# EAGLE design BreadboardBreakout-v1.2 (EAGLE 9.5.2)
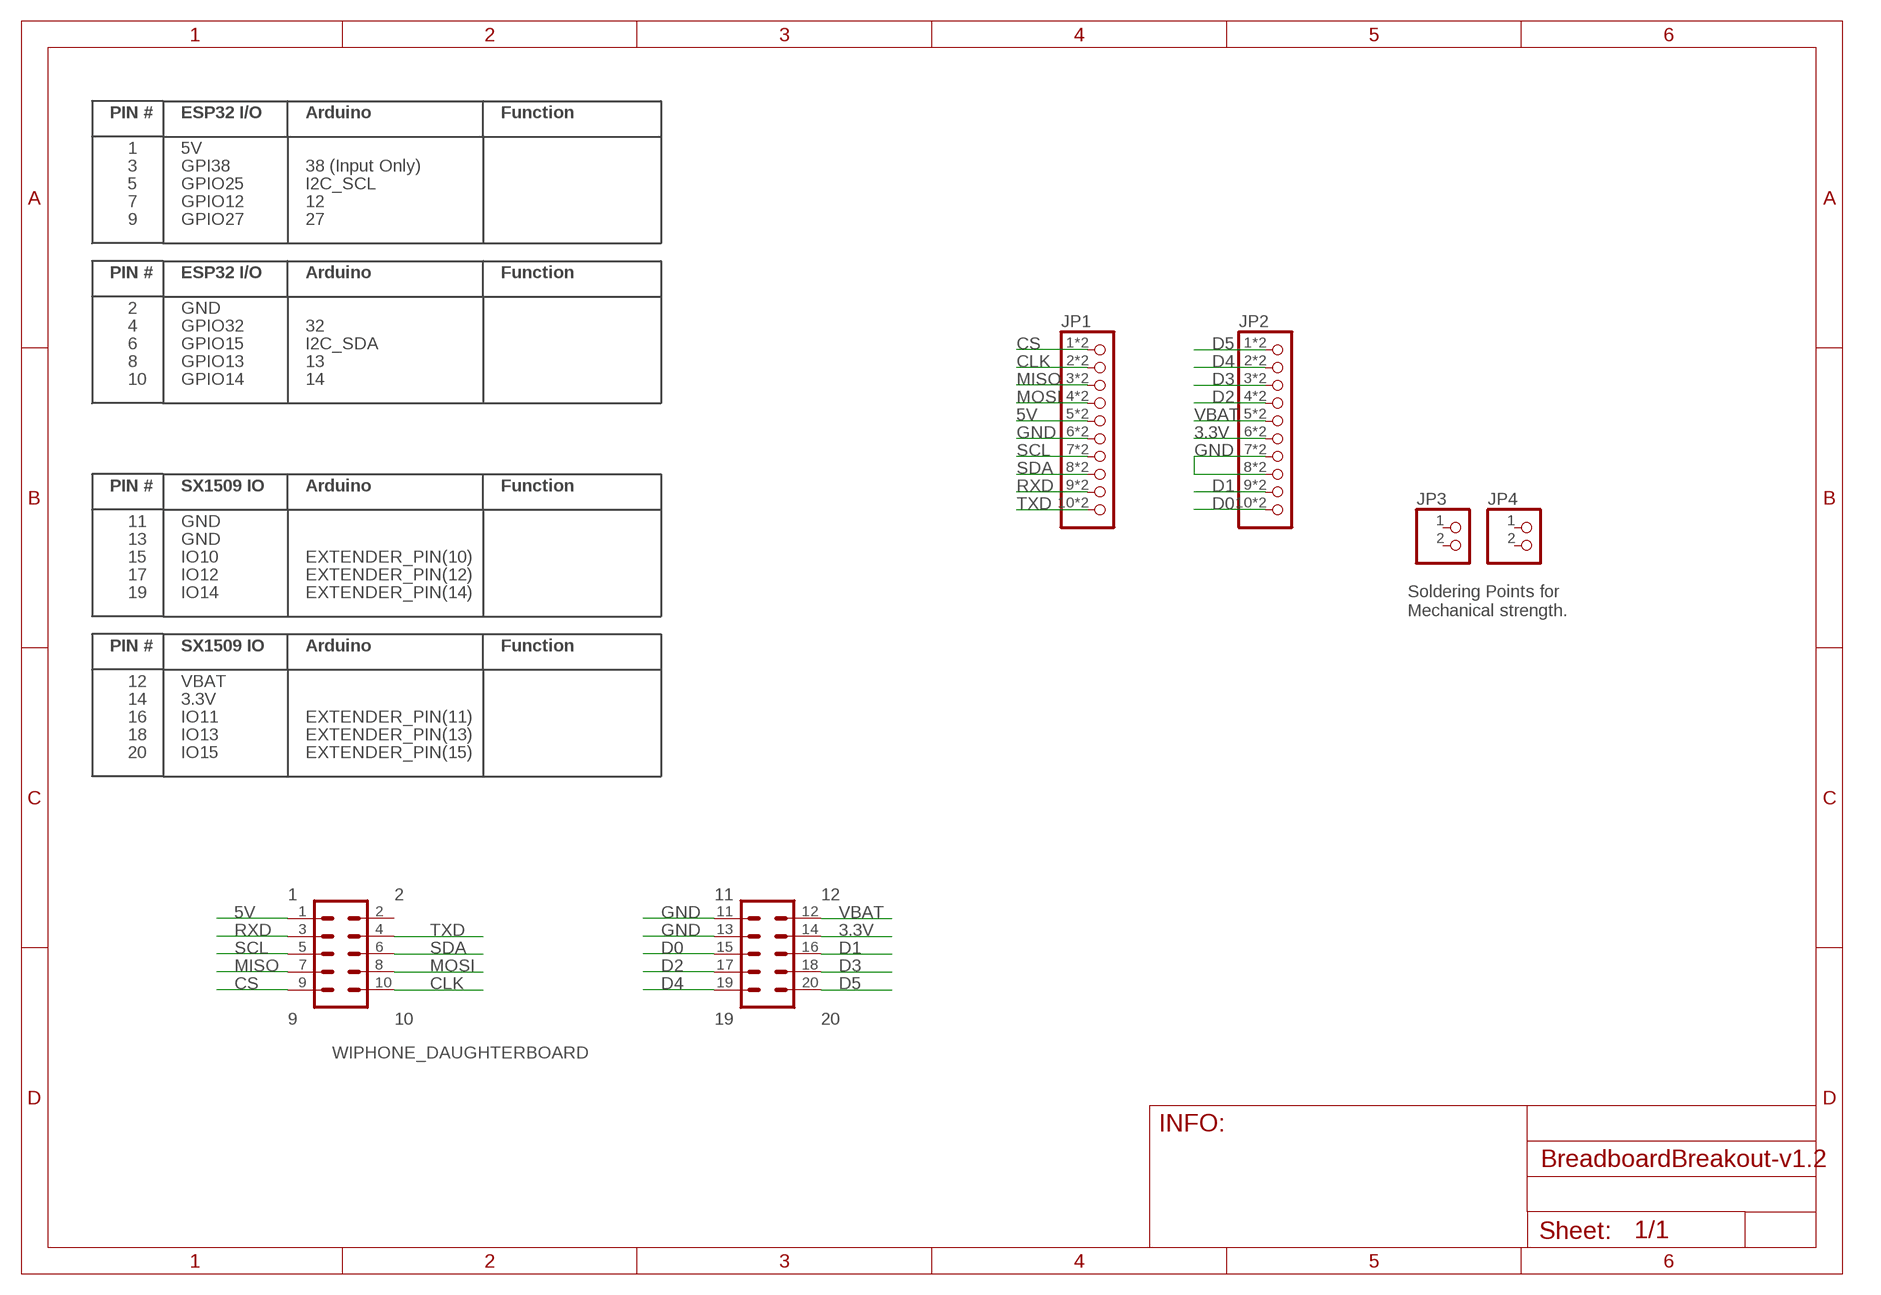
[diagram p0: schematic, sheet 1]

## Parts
JP1  PINHD-1X10_TH/SMD  [1X10TH/SMD]
JP2  PINHD-1X10_TH/SMD  [1X10TH/SMD]
JP3  PINHD-1X2_EXT  [1X02TH/EXT]
JP4  PINHD-1X2_EXT  [1X02TH/EXT]
WIPHONE_DAUGHTERBOARD-FOOTPRINT1  WIPHONE_DAUGHTERBOARD  [WIPHONE_DAUGHTERBOARD]

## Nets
3.3V: JP2.6 JP2.6P WIPHONE_DAUGHTERBOARD-FOOTPRINT1.14
5V: JP1.5 JP1.5P WIPHONE_DAUGHTERBOARD-FOOTPRINT1.1
CLK: JP1.2 JP1.2P WIPHONE_DAUGHTERBOARD-FOOTPRINT1.10
CS: JP1.1 JP1.1P WIPHONE_DAUGHTERBOARD-FOOTPRINT1.9
D0: JP2.10 JP2.10P WIPHONE_DAUGHTERBOARD-FOOTPRINT1.15
D1: JP2.9 JP2.9P WIPHONE_DAUGHTERBOARD-FOOTPRINT1.16
D2: JP2.4 JP2.4P WIPHONE_DAUGHTERBOARD-FOOTPRINT1.17
D3: JP2.3 JP2.3P WIPHONE_DAUGHTERBOARD-FOOTPRINT1.18
D4: JP2.2 JP2.2P WIPHONE_DAUGHTERBOARD-FOOTPRINT1.19
D5: JP2.1 JP2.1P WIPHONE_DAUGHTERBOARD-FOOTPRINT1.20
GND: JP1.6 JP1.6P JP2.7 JP2.7P JP2.8 JP2.8P WIPHONE_DAUGHTERBOARD-FOOTPRINT1.11 WIPHONE_DAUGHTERBOARD-FOOTPRINT1.13
MISO: JP1.3 JP1.3P WIPHONE_DAUGHTERBOARD-FOOTPRINT1.7
MOSI: JP1.4 JP1.4P WIPHONE_DAUGHTERBOARD-FOOTPRINT1.8
RXD: JP1.9 JP1.9P WIPHONE_DAUGHTERBOARD-FOOTPRINT1.3
SCL: JP1.7 JP1.7P WIPHONE_DAUGHTERBOARD-FOOTPRINT1.5
SDA: JP1.8 JP1.8P WIPHONE_DAUGHTERBOARD-FOOTPRINT1.6
TXD: JP1.10 JP1.10P WIPHONE_DAUGHTERBOARD-FOOTPRINT1.4
VBAT: JP2.5 JP2.5P WIPHONE_DAUGHTERBOARD-FOOTPRINT1.12
Unconnected: JP3.1 JP3.2 JP4.1 JP4.2

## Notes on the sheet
- Soldering Points for 
  Mechanical strength.

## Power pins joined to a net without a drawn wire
2: WIPHONE_DAUGHTERBOARD-FOOTPRINT1.2

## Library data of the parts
JP1 JP2 = WiPhone:PINHD-1X10: PIN HEADER
JP3 JP4 = WiPhone:PINHD-1X2: PIN HEADER
WIPHONE_DAUGHTERBOARD-FOOTPRINT1 = WiPhone:WIPHONE_DAUGHTERBOARD

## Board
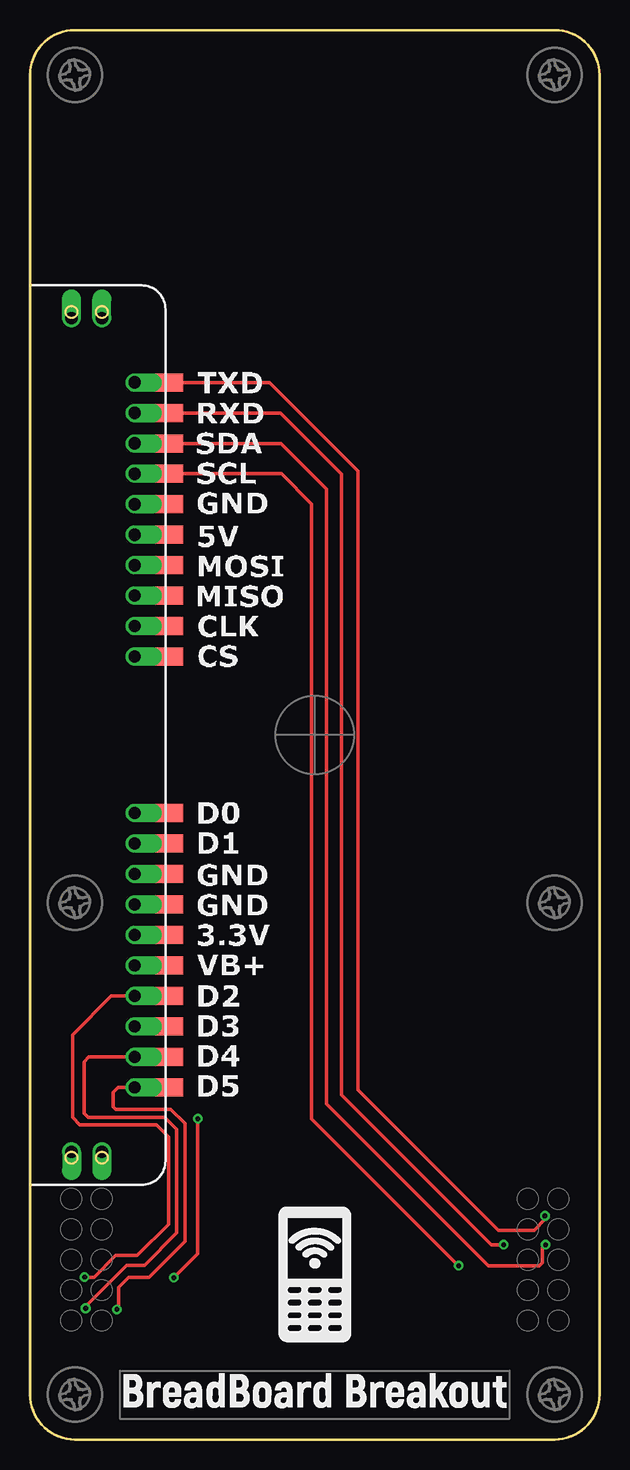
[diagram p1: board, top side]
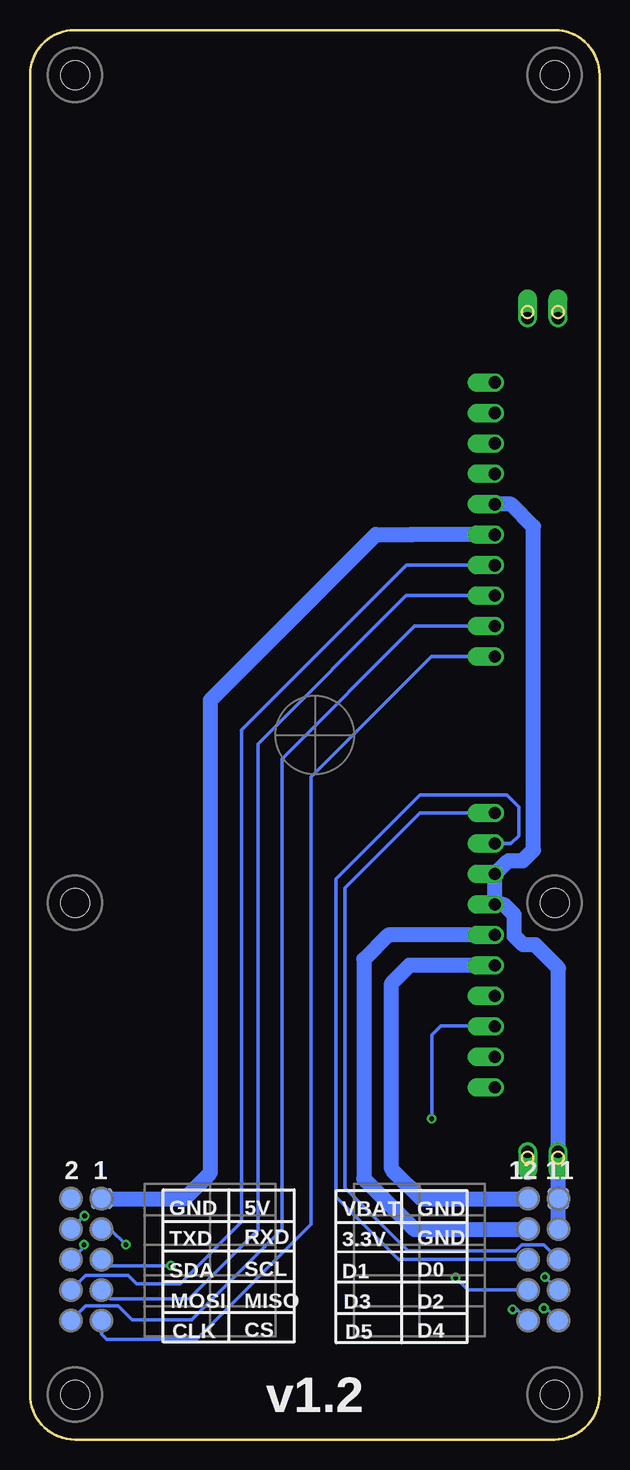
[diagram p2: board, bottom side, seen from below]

Size 47.5 x 117.5 mm. Coordinates in mm from the lower left corner, seen from the top.
Copper layers (1*16): Top 0.035mm / dielectric 1.5mm / Bottom 0.035mm
Design rules "2LDaughterBoards": minimum track width 6mil, minimum drill 6mil, track to track 8mil, track to pad 8mil, pad to pad 8mil, via to via 8mil, smd to smd 0mil, copper to edge 16mil, drill to drill 6mil, minimum pad ring 10mil, minimum via ring 8mil, stop-mask expansion 4mil, vias tented up to drill 25mil, thermal gap 10mil

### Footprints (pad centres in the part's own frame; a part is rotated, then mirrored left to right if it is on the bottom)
1X10TH/SMD = drill 1.016 pad 1.5 offset: 1 0,-11.43; 2 0,-8.89; 3 0,-6.35; 4 0,-3.81; 5 0,-1.27; 6 0,1.27; 7 0,3.81; 8 0,6.35; 9 0,8.89; 10 0,11.43 | smd 3 x 1.5: 1P 2.57,-11.43; 2P 2.57,-8.89; 3P 2.57,-6.35; 4P 2.57,-3.81; 5P 2.57,-1.27; 6P 2.57,1.27; 7P 2.57,3.81; 8P 2.57,6.35; 9P 2.57,8.89; 10P 2.57,11.43
1X02TH/EXT = drill 1.016 pad 1.575 offset: 1 0,-2.54; 2 0,0
WIPHONE_DAUGHTERBOARD = smd 1.75 x 1.75 bottom: 1 17.78,-38.66; 2 20.32,-38.66; 3 17.78,-41.2; 4 20.32,-41.2; 5 17.78,-43.74; 6 20.32,-43.74; 7 17.78,-46.28; 8 20.32,-46.28; 9 17.78,-48.82; 10 20.32,-48.82; 11 -20.32,-38.66; 12 -17.78,-38.66; 13 -20.32,-41.2; 14 -17.78,-41.2; 15 -20.32,-43.74; 16 -17.78,-43.74; 17 -20.32,-46.28; 18 -17.78,-46.28; 19 -20.32,-48.82; 20 -17.78,-48.82 | hole 2.4: 20,-54.991; -20,-54.991; 20,-13.991; 20,55.009; -20,55.009; -20,-13.991

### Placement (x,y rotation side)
JP1  8.72,76.69 0 top
JP2  8.72,40.79 0 top
JP3  3.46,93.49 90 top
JP4  6,23.99 270 top
WIPHONE_DAUGHTERBOARD-FOOTPRINT1  23.75,58.74 0 top

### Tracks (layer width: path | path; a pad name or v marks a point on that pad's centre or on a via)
3.3V
  Top 1.27: JP2.6P JP2.6
  Bottom 1.27: JP2.6 17.63,42.06 19.65,40.04 19.65,21.74 15.42,17.52 5.99,17.52 WIPHONE_DAUGHTERBOARD-FOOTPRINT1.14
5V
  Top 1.27: JP1.5P JP1.5
  Bottom 1.27: JP1.5 15.67,75.42 15.69,75.44 18.65,75.44 32.45,61.64 32.45,22.24 34.62,20.07 34.64,20.08 WIPHONE_DAUGHTERBOARD-FOOTPRINT1.1
CLK
  Top 0.305: JP1.2 JP1.2P
  Bottom 0.305: JP1.2 15.44,67.8 26.5,56.74 26.5,17.53 34.04,9.99 39,9.99 40.16,11.15 42.84,11.15 WIPHONE_DAUGHTERBOARD-FOOTPRINT1.10
CS
  Top 0.305: JP1.1 JP1.1P
  Bottom 0.305: JP1.1 14.03,65.26 24.05,55.24 24.05,17.94 33.62,8.37 41.12,8.37 41.53,8.77 WIPHONE_DAUGHTERBOARD-FOOTPRINT1.9
D0
  Top 0.305: JP2.10P JP2.10
  Bottom 0.305: JP2.10 14.98,52.22 15,52.24 21.25,45.99 21.25,20.99 16,15.74 6.97,15.74 6.48,16.23 4.66,16.23 WIPHONE_DAUGHTERBOARD-FOOTPRINT1.15
D1
  Top 1.27: JP2.9P JP2.9
  Bottom 0.305: WIPHONE_DAUGHTERBOARD-FOOTPRINT1.16 16.73,15 16.74,14.99 22,20.24 22,46.74 15,53.74 7.75,53.74 6.75,52.74 6.75,50.32 7.39,49.68 JP2.9
D2  (via drill 0.41)
  Top 0.305: v4.55,13.54 5.35,13.54 7.15,15.34 8.95,15.34 11.55,17.94 11.55,25.24 10.55,26.24 4.15,26.24 3.55,26.84 3.55,33.74 6.79,36.98 JP2.4 JP2.4P
  Bottom 0.305: WIPHONE_DAUGHTERBOARD-FOOTPRINT1.17 4.51,13.54 v4.55,13.54
D3  (via drill 0.41)
  Top 0.305: v12,13.49 14,15.49 v14,26.74 | JP2.3 JP2.3P
  Bottom 0.305: v12,13.49 10.95,12.45 10.94,12.46 WIPHONE_DAUGHTERBOARD-FOOTPRINT1.18 | v14,26.74 14,33.74 13.25,34.49 8.77,34.49 JP2.3
D4  (via drill 0.41)
  Top 0.305: JP2.2 4.91,31.9 4.51,31.5 4.51,27.18 4.85,26.84 11.25,26.84 12.25,25.84 12.25,17.24 9.55,14.54 8.05,14.54 4.55,11.04 v4.65,10.94
  Top 1.27: JP2.2P JP2.2
  Bottom 0.305: WIPHONE_DAUGHTERBOARD-FOOTPRINT1.19 4.45,10.94 v4.65,10.94
D5  (via drill 0.41)
  Top 0.305: JP2.1 7.37,29.36 6.95,28.94 6.95,27.74 7.15,27.54 11.75,27.54 12.95,26.34 12.95,16.54 9.95,13.54 8.25,13.54 7.4,12.69 7.4,10.99 v7.25,10.84
  Top 1.27: JP2.1P JP2.1
  Bottom 0.305: WIPHONE_DAUGHTERBOARD-FOOTPRINT1.20 6.89,10.84 v7.25,10.84
GND
  Top 1.27: JP2.7P JP2.7 | JP2.8P JP2.8 | JP1.6P JP1.6
  Bottom 1.27: WIPHONE_DAUGHTERBOARD-FOOTPRINT1.13 WIPHONE_DAUGHTERBOARD-FOOTPRINT1.11 3.43,39.31 5.35,41.23 6.37,41.23 7.11,41.97 7.11,43.73 7.98,44.6 JP2.7 JP2.8 7.59,48.27 6.39,48.27 5.52,49.14 5.52,76.1 7.37,77.96 JP1.6
MISO
  Top 0.305: JP1.3 JP1.3P
  Bottom 0.305: JP1.3 16.15,70.34 28.5,57.99 28.5,17.49 34.25,11.74 40.81,11.74 WIPHONE_DAUGHTERBOARD-FOOTPRINT1.7
MOSI
  Top 0.305: JP1.4 JP1.4P
  Bottom 0.305: JP1.4 16.11,72.88 29.85,59.14 29.85,18.14 35,12.99 38.59,12.99 39.29,13.69 42.84,13.69 WIPHONE_DAUGHTERBOARD-FOOTPRINT1.8
RXD  (via drill 0.41)
  Top 0.305: v39.5,16.24 38.5,16.24 26,28.74 26,80.49 20.91,85.58 JP1.9P JP1.9
  Bottom 0.305: WIPHONE_DAUGHTERBOARD-FOOTPRINT1.3 40.8,17.54 v39.5,16.24
SCL  (via drill 0.41)
  Top 0.305: v35.75,14.49 23.5,26.74 23.5,77.99 20.99,80.5 JP1.7P JP1.7
  Bottom 0.305: WIPHONE_DAUGHTERBOARD-FOOTPRINT1.5 41.02,14.49 v35.75,14.49
SDA  (via drill 0.41)
  Top 0.305: v43,16.24 42.75,15.99 42.75,14.74 42.5,14.49 38.25,14.49 24.75,27.99 24.75,79.24 20.95,83.04 JP1.8P JP1.8
  Bottom 0.305: WIPHONE_DAUGHTERBOARD-FOOTPRINT1.6 43,16.07 v43,16.24
TXD  (via drill 0.41)
  Top 0.305: 10.65,88.12 19.97,88.12 27.35,80.74 27.35,29.14 39.05,17.44 42.05,17.44 42.95,18.34 v42.95,18.64 | JP1.10 9.35,88.12
  Top 1.27: JP1.10P 10.65,88.12 9.35,88.12
  Bottom 0.305: WIPHONE_DAUGHTERBOARD-FOOTPRINT1.4 42.97,18.64 v42.95,18.64
VBAT
  Top 1.27: JP2.5P JP2.5
  Bottom 1.27: JP2.5 15.87,39.52 17.35,38.04 17.35,22.54 14.87,20.07 5.98,20.07 WIPHONE_DAUGHTERBOARD-FOOTPRINT1.12

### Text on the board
bPlace: v1.2
bNames: GND | VBAT | 5V | GND | RXD | GND | 3.3V | TXD | D0 | D1 | SCL | SDA | D2 | D3 | MISO | MOSI | D4 | D5 | CS | CLK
